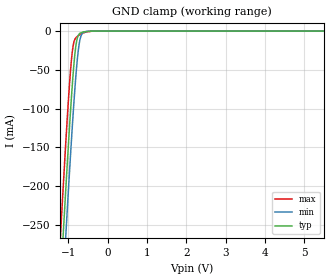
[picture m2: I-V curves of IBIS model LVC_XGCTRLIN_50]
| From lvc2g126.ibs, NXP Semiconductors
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|   Model LVC_XGCTRLIN_50
[Model]   LVC_XGCTRLIN_50
Model_type   Input
Vinl =   1.5V
Vinh =   3.5V
C_comp   2.8549pF   1.9655pF   3.9020pF
|Ambient temperature:   25   85   -40
[Temperature Range]   50   105   -10
[Voltage Range]   5.0V   4.5V   5.5V
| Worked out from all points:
|   GND clamp passes 1 mA (typ) near -0.59 V on its own axis
|Process Range   nominal   slow   fast
[GND_clamp]
| voltage   I(typ)   I(min)   I(max)
-5.5V     -4.553A    -4.607A    -4.5A
-1.208V   -334.3mA   -394.9mA   -272.4mA
-1.186V   -314mA     -374.6mA   -252.2mA
-1.142V   -273.9mA   -334.3mA   -212.3mA
-1.12V    -254.1mA   -314.4mA   -192.7mA
-1.054V   -195.5mA   -255.2mA   -135.3mA
-966mV    -121.2mA   -178.9mA   -65.98mA
-900mV    -70.86mA   -124.8mA   -27.22mA
-790mV    -13.47mA   -47.2mA    -7.678mA
-680mV    -2.175mA   -6.549mA   -3.932mA
-378mV    -104.7uA   -93.25uA   -115.5uA
5.5V      0A         0A         0A
